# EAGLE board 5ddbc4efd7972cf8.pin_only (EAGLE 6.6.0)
REV: B

Size 45.72 x 49.53 mm. Coordinates in mm from the lower left corner, seen from the top.
Outline: 0,0 45.72,0 45.72,46.99 arc90 43.18,49.53 2.54,49.53 arc90 0,46.99 0,11.18 1.27,11.18 1.27,7.62 0,7.62 0,0
Copper layers (1*16): Top 0.035mm / dielectric 1.5mm / Bottom 0.035mm
Design rules "adafruit *": minimum track width 8mil, minimum drill 15.5mil, track to track 8mil, track to pad 8mil, pad to pad 8mil, via to via 8mil, smd to smd 8mil, copper to edge 10mil, drill to drill 8mil, minimum pad ring 10mil, minimum via ring 8mil, stop-mask expansion 2mil, vias tented up to drill 20mil, thermal gap 10mil
tRestrict: area 13.7,34.7 to 14.2,34.8; area 13.7,21.6 to 14.2,21.7; area 19.9,13.5 to 20.1,14; area 21.8,43.4 to 22,43.9

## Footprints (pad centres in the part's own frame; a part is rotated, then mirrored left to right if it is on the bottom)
0805-NO = smd 1.3 x 1.5: 1 -0.95,0; 2 0.95,0
C1210 = smd 1.6 x 2.7: 1 -1.4,0; 2 1.4,0
RESPACK_4X0603 = smd 0.45 x 0.9: 1 -1.3,-0.85; 2 -0.4,-0.85; 3 0.4,-0.85; 4 1.3,-0.85; 5 1.3,0.85; 6 0.4,0.85; 7 -0.4,0.85; 8 -1.3,0.85
CHIPLED_0805_NOOUTLINE = smd 1.2 x 1.2: A 0,-1.05; C 0,1.05
JSTPH2 = smd 1 x 4.6: 1 -1,-3.7; 2 1,-3.7 | smd 1.6 x 3.4: NC1 -3.4,1.5; NC2 3.4,1.5
SOD-123 = smd 1.4 x 1.4: A 1.85,0; C -1.85,0
SOT363 = smd 0.5 x 0.5: 1 -0.75,-0.9; 3 0.75,-0.9; 4 0.75,0.9; 6 -0.75,0.9 | smd 0.4 x 0.5: 2 0,-0.9; 5 0,0.9
SOD-323 = smd 1.35 x 0.8: A 1.27,0; C -1.27,0
FIDUCIAL_1MM = smd 1 x 1: 1 0,0
SOLDERJUMPER_ARROW_NOPASTE = smd 0.762 x 1.524: 1 -1.016,0; 2 1.016,0
TSSOP14 = smd 0.35 x 0.9: 1 -1.95,-2.925; 2 -1.3,-2.925; 3 -0.65,-2.925; 4 0,-2.925; 5 0.65,-2.925; 6 1.3,-2.925; 7 1.95,-2.925; 8 1.95,2.925; 9 1.3,2.925; 10 0.65,2.925; 11 0,2.925; 12 -0.65,2.925; 13 -1.3,2.925; 14 -1.95,2.925
1X18_ROUND70 = drill 1 pad 1.778: 1 -21.59,0; 2 -19.05,0; 3 -16.51,0; 4 -13.97,0; 5 -11.43,0; 6 -8.89,0; 7 -6.35,0; 8 -3.81,0; 9 -1.27,0; 10 1.27,0; 11 3.81,0; 12 6.35,0; 13 8.89,0; 14 11.43,0; 15 13.97,0; 16 16.51,0; 17 19.05,0; 18 21.59,0
1X02_ROUND = drill 1 pad 1.778: 1 -1.27,0; 2 1.27,0
_0805MP = smd 1.2 x 1.3: 1 -1.016,0; 2 1.016,0
SOT23-WIDE = smd 1 x 1.2: 1 -0.95,-1; 2 0.95,-1; 3 0,1
BTN_KMR2_4.6X2.8 = smd 0.9 x 1: A 2.05,0.8; A' -2.05,0.8; B 2.05,-0.8; B' -2.05,-0.8
TP11R = smd 1.1 x 1.1: TP 0,0
SIM5320 = smd 1.8 x 0.6: 1 -15,9.5; 2 -15,8.5; 3 -15,7.5; 4 -15,6.5; 5 -15,5.5; 6 -15,4.5; 7 -15,3.5; 8 -15,2.5; 9 -15,1.5; 10 -15,0.5; 11 -15,-0.5; 12 -15,-1.5; 13 -15,-2.5; 14 -15,-3.5; 15 -15,-4.5; 16 -15,-5.5; 17 -15,-6.5; 18 -15,-7.5; 19 -15,-8.5; 20 -15,-9.5; 41 15,-9.5; 42 15,-8.5; 43 15,-7.5; 44 15,-6.5; 45 15,-5.5; 46 15,-4.5; 47 15,-3.5; 48 15,-2.5; 49 15,-1.5; 50 15,-0.5; 51 15,0.5; 52 15,1.5; 53 15,2.5; 54 15,3.5; 55 15,4.5; 56 15,5.5; 57 15,6.5; 58 15,7.5; 59 15,8.5; 60 15,9.5 | smd 0.6 x 1.8: 21 -9.5,-15; 22 -8.5,-15; 23 -7.5,-15; 24 -6.5,-15; 25 -5.5,-15; 26 -4.5,-15; 27 -3.5,-15; 28 -2.5,-15; 29 -1.5,-15; 30 -0.5,-15; 31 0.5,-15; 32 1.5,-15; 33 2.5,-15; 34 3.5,-15; 35 4.5,-15; 36 5.5,-15; 37 6.5,-15; 38 7.5,-15; 39 8.5,-15; 40 9.5,-15; 61 9.5,15; 62 8.5,15; 63 7.5,15; 64 6.5,15; 65 5.5,15; 66 4.5,15; 67 3.5,15; 68 2.5,15; 69 1.5,15; 70 0.5,15; 71 -0.5,15; 72 -1.5,15; 73 -2.5,15; 74 -3.5,15; 75 -4.5,15; 76 -5.5,15; 77 -6.5,15; 78 -7.5,15; 79 -8.5,15; 80 -9.5,15
SOT23-5 = smd 0.55 x 1.2: 1 -0.95,-1.3; 2 0,-1.3; 3 0.95,-1.3; 4 0.95,1.3; 5 -0.95,1.3
MOUNTINGHOLE_2.5_PLATED = drill 2.5 pad 3.2: P$1 0,0
SMA_EDGELAUNCH_UFL = smd 4.064 x 1.524: GND@1 2.032,-2.54; GND@2 2.032,2.54 | smd 4.064 x 1.524 bottom: GND@3 2.032,2.54; GND@4 2.032,-2.54 | smd 2.032 x 1.016: P 3.048,0
4UCONN_20329 = smd 1 x 2: BASE@1 -0.75,-2; BASE@2 0.75,-2 | smd 0.4 x 1.35: D+ 0,0.775; D- -0.65,0.775; GND 1.3,0.775; ID 0.65,0.775; VBUS -1.3,0.775 | drill 0.7 offset: SPRT@1 -3.3,0.9; SPRT@2 3.3,0.9 | drill 0.6 pad 2.5 square: SPRT@3 -3.6,-1.9; SPRT@4 3.6,-1.9 | hole 0.7: -1.95,0; 1.95,0
U.FL = smd 2.2 x 1.05: 1 0,1.375; 2 0,-1.375 | smd 0.8 x 1: 3 1.525,0
4UCONN_18510 = smd 1.5 x 2.5: 1-GND 2.8,-3.3; 2-TIP 9.3,3.4; 3-OUTER_SLEEVE 5.5,-3.3 | smd 1.5 x 3.4: 4-INNER_SLEEVE 2.8,2.9 | hole 1.3: 10.5,0
C707_10M006_512_2 = smd 1.7 x 1.3: C1 -12.85,-3.915; C2 -12.85,-1.375; C3 -12.85,1.165; C5 12.85,-3.915; C6 12.85,-1.375; C7 12.85,1.165

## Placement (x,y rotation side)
C1  10µF  [0805-NO]  7.37,28.07 270 top
C2  100uF  [C1210]  38.48,46.74 180 top
C3  33pF  [0805-NO]  11.18,21.46 0 top
C4  33pF  [0805-NO]  12.57,16 270 top
C5  10pF  [0805-NO]  11.67,42.18 0 top
C6  33pF  [0805-NO]  11.76,40.08 0 top
C7  100uF  [C1210]  11.05,35.69 270 top
C8  10pF  [0805-NO]  10.54,16 270 top
C9  10uF  [0805-NO]  35.18,46.74 90 top
C10  33pF  [0805-NO]  10.41,19.68 180 top
C11  10uF  [0805-NO]  6.22,13.84 0 top
C14  33pF  [RESPACK_4X0603]  34.04,6.73 90 top
C15  10pF  [RESPACK_4X0603]  37.21,6.73 90 top
C16  33pF  [RESPACK_4X0603]  42.93,11.43 0 top
C17  10pF  [RESPACK_4X0603]  42.93,7.37 0 top
CHRG  ORANGE  [CHIPLED_0805_NOOUTLINE]  2.16,32.4 270 top
CN2  JSTPH  [JSTPH2]  3.56,39.88 90 top
D1  MMSZ5231BT1G  [SOD-123]  10.79,44.7 0 top
D2  SMF05C  [SOT363]  37.21,10.79 180 top
D3  1N4148  [SOD-323]  17.78,7.75 90 top
D4  1N4148  [SOD-323]  13.97,6.99 90 top
D5  1N4148  [SOD-323]  16,7.75 90 top
D6  1N4148  [SOD-323]  19.56,7.75 90 top
DONE  GREEN  [CHIPLED_0805_NOOUTLINE]  2.17,34.24 90 top
FID1  FIDUCIAL""  [FIDUCIAL_1MM]  40.51,28.57 0 top
FID2  FIDUCIAL""  [FIDUCIAL_1MM]  2.16,39.5 0 top
FID3  FIDUCIAL""  [FIDUCIAL_1MM]  5.59,9.53 0 top
FID4  FIDUCIAL""  [FIDUCIAL_1MM]  6.1,47.62 0 bottom
FID5  FIDUCIAL""  [FIDUCIAL_1MM]  28.57,25.02 0 bottom
GPSBIAS  [SOLDERJUMPER_ARROW_NOPASTE]  7.11,18.41 90 top
IC1  74VHCT125PW  [TSSOP14]  29.46,8.13 180 top
JP1  [1X18_ROUND70]  22.86,1.78 0 top
JP2  [1X02_ROUND]  25.4,46.99 270 top
L2  33nH  [_0805MP]  7.62,21.46 0 top
NETSTAT  RED  [CHIPLED_0805_NOOUTLINE]  29.46,47.62 0 top
PWRSTAT  GREEN  [CHIPLED_0805_NOOUTLINE]  33.53,47.62 0 top
Q2  bss138  [SOT23-WIDE]  24.51,9.65 180 top
R1  470  [0805-NO]  5.84,32.26 0 top
R2  1K  [0805-NO]  5.86,34.16 0 top
R3  2K  [0805-NO]  10.29,27.56 180 top
R4  1K  [0805-NO]  31.5,46.61 270 top
R5  1K  [0805-NO]  27.81,46.61 270 top
R6  2K  [0805-NO]  13.97,10.79 90 top
R8  10K  [0805-NO]  23.24,6.86 180 top
SW1  KMR2  [BTN_KMR2_4.6X2.8]  10.79,47.62 0 top
TP1  TPTP11R  [TP11R]  35.56,40.39 0 bottom
U1  SIM5320  [SIM5320]  28.96,28.7 90 top
U2  MCP73831T-2ACI/OT  [SOT23-5]  10.79,30.73 180 top
U$21  [ADAFRUIT_2.5MM]  9.02,23.62 90 top
U$25  [PCBFEAT-REV-040]  2.29,25.53 0 bottom
U$26  [FONA_LOGO]  19.94,32.38 0 bottom
U$33  MOUNTINGHOLE2.5  [MOUNTINGHOLE_2.5_PLATED]  43.18,46.99 90 top
U$34  MOUNTINGHOLE2.5  [MOUNTINGHOLE_2.5_PLATED]  2.54,46.99 90 top
U$36  [ADAFRUIT_5MM]  14.86,44.07 0 bottom
U$42  [ADAFRUIT_TEXT_20MM]  37.85,10.16 90 bottom
X1  uFL  [SMA_EDGELAUNCH_UFL]  20.45,49.28 270 top
X2  MicroB  [4UCONN_20329]  4.19,25.4 270 top
X3  uFL  [U.FL]  2.16,17.4 0 top
X4  4UCONN_18510  [4UCONN_18510]  0.13,9.4 0 top
X6  SIM_LOCKAMPHENOL  [C707_10M006_512_2]  28.45,24.77 270 bottom

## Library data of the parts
C1 C3-C6 C8-C11 C14-C17 CHRG CN2 D1-D3 D6 DONE JP1 JP2 L2 NETSTAT PWRSTAT Q2 R1-R6 R8 SW1 U1 U2 U$21 U$25 U$26 U$36 U$42 X1-X4 = microbuilder
C2 C7 = rcl
D4 D5 = microbuilder; COMPANY: ADAFRUIT INDUSTRIES; DRAWN: KTOWN; REV: A
FID1-FID5 GPSBIAS U$33 U$34 = microbuilder; BOM: EXCLUDE
IC1 = 74xx-us
TP1 = testpad
X6 = microbuilder; OC_FARNELL: unknown; OC_NEWARK: unknown

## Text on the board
tPlace: PWR / Key | Net | PWR | Cell / ANT | bias | GPSANT | in | out | SPKR | 5V | Bat | Gnd | Vio | Rst | RX | TX | RTS | DTR | CTS | Key | RI | PS | NS | + | Mic | - | + | -
bPlace: SDA | SCL | FONA 3G/GSM+GPS | 2.8V | Data/Voice/SMS | 3G Cell-Phone | with GPS | 50Ω Passive GPS / Short bias jumper / for active GPS ant. | CTIA Headset / TRRS: LR-M | 3.7V LiPoly | Req. during use | 0.5A USB Charging | Vio: I/O Level 3-5VDC

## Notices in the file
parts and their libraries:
microbuilder: This work is placed in the public domain, and may be freely used for commercial and non-commercial work with the following conditions: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
